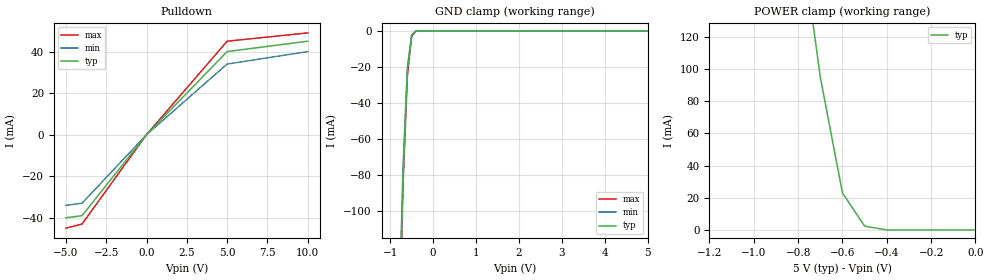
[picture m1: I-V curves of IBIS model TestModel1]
[IBIS Ver]   3.2
[File Name]   bug53.ibs
[File Rev]   0.0
[Date]   05-January-2001
[Source]   File created from specification
[Notes]   Using the IBISCHK3 v3.2.6 parser, the following file
   will generate a single warning regarding the lack of
   a [Pullup] section.  This warning does not appear in
   the v.3.2.5 parser's output.
[Disclaimer]
   (C) Copyright 2001 Intel Corp.
   All rights reserved
   This model is for demonstration purposes only,
[Component]   GENERIC_IBIS
[Manufacturer]   Intel Corp.
[Package]
|   typ   min   max
R_pkg   6.0mO   5.0mO   7.0mO
L_pkg   5.0nH   2.0nH   8.0nH
C_pkg   1.0pF   0.5pF   1.5pF
[Pin]   signal_name   model_name   R_pin   L_pin   C_pin
   1   TestSignal1   TestModel1
| Models and submodels in the file (1): TestModel1 (I/O_open_drain)
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[Model]   TestModel1
Model_type   I/O_open_drain
Polarity   Non-Inverting
Vinl = 800mV
Vinh = 2.0V
Cref = 10.0pF
Vref = 0.0
Vmeas = 0.4
C_comp   5.00pF   4.00pF   6.00pF
[Temperature Range]   27.00   100.00   0.00
[Voltage Range]   5.0V   4.75V   5.25V
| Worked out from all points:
|   slope of the pulldown table from 0 to 0.75 V, typ, clamps not added: 125 ohm
|   GND clamp passes 1 mA (typ) near -0.44 V on its own axis
|   POWER clamp passes 1 mA (typ) near -0.44 V on its own axis
[Pulldown]
| voltage   I(typ)   I(min)   I(max)
-5V       -40mA      -34mA      -45mA
-4V       -39mA      -33mA      -43mA
0V        0A         0A         0A
5V        40mA       34mA       45mA
10V       45mA       40mA       49mA
[GND Clamp]
| voltage   I(typ)   I(min)   I(max)
-5V       -3.9A      -3.8A      -4A
-700mV    -80mA      -75mA      -85mA
-600mV    -22mA      -20mA      -25mA
-500mV    -2.4mA     -2mA       -2.9mA
-400mV    0A         0A         0A
5V        0A         0A         0A
[Power Clamp]
| voltage   I(typ)   I(min)   I(max)
-5V       4.45A      NA         NA
-700mV    95mA       NA         NA
-600mV    23mA       NA         NA
-500mV    2.4mA      NA         NA
-400mV    0A         NA         NA
0V        0A         NA         NA
[Ramp]
|variable   typ   min   max
dV/dt_r   2.20/1.06n   1.92/1.28n   2.49/650p
dV/dt_f   2.46/1.21n   2.21/1.54n   2.70/770p
R_load = 300ohms
